| TEXAS INSTRUMENTS INCORPORATED
| Standard Linear and Logic Group
| IBIS Model of SN74AHC139
| DUAL 2-LINE TO 4-LINE DECODERS/DEMULTIPLEXERS
| This file contains package information for the following:
|  SOIC 16-pin (D) package as [Component] AHC139_D
|  SSOP 16-pin (DB) package as [Component] AHC139_DB
|  TVSOP 16-pin (DGV) package as [Component] AHC139_DGV
|  PDIP 16-pin (N) package as [Component] AHC139_N
|  SOP 16-pin (NS) package as [Component] AHC139_NS
|  TSSOP 16-pin (PW) package as [Component] AHC139_PW
|  QFN 16-pin (RGY) package as [Component] AHC139_RGY
| This device can be powered at the following Vccs:
|  5 volt Vcc
|  3.3 volt Vcc
| This file provides unique models under the [Model Selector] for each Vcc.
| For operation at a specific Vcc, select the appropriate model after each
| [Model Selector] keyword.
[IBIS Ver]   3.2
[Comment char]  |_char
[File Name]   sn74ahc139.ibs
[File Rev]   1.1 | X_die
[Date]   May 23, 2005
[Source]   Data created from TI-SPICE simulations at TI-SLL.
[Notes]   The following is an IBIS list for the AHC139.
   Please contact sllibis@ti.com with questions and
   comments concerning SLL IBIS models.
   This IBIS model is created from a BA (back annotated netlist)
   - FILE REV HISTORY
   - 1.1 Release IBIS file on 06/20/05
   - C_comp values are taken at a different test condition
   than the data sheet.
   - Power clamp data deleted as there is no power-clamp diode.
[Disclaimer] Property of Texas Instruments Incorporated.  Unauthorized
   reproduction and/or distribution is strictly prohibited.
   This product is protected under copyright law.
   Created  2005, (C) Copyright  2005, Texas Instruments
   Incorporated, All Rights Reserved
   UNLESS THERE IS A SIGNED, WRITTEN AGREEMENT TO THE
   CONTRARY, TEXAS INSTRUMENTS (TI) IS PROVIDING THE IBIS
   MODELS  AND WITHOUT ANY WARRANTY, EXPRESSED OR
   IMPLIED.  TI assumes no liability for:
   1) the accuracy of the IBIS models provided to your
   company;
   2) the proper functioning of these IBIS Models in your
   design or for any resulting applications; or
   3) infringement of patents, copyrights or intellectual
   property rights resulting from your use of these IBIS
   models.
   TI provides IBIS Models as a service to our customers.
   You and your company shall not distribute, sell or give
   these models to anyone else without prior written
   permission from TI.
   TI reserves the right to make changes to our products or
   to discontinue any semiconductor product or service
   without notice, and advises our customers to obtain the
   latest version of relevant information to verify, before
   placing orders, that the information being relied on is
   current.
   Please be aware that your receipt and use of the IBIS
   information provided shall serve as acceptance of these
   terms and conditions.  If you do not accept these terms,
   you should return or destroy the IBIS models and any
   other accompanying information immediately.
| Component ahc139_D 16-pin SOIC
[Component]   ahc139_D
[Manufacturer]   Texas Instruments, Inc.
[Package]
|   typ   min   max
R_pkg   3.900e-02   2.800e-02   4.900e-02
L_pkg   3.453e-09   2.350e-09   4.375e-09
C_pkg   5.210e-13   2.540e-13   7.080e-13
[Pin]   signal_name   model_name   R_pin   L_pin   C_pin
1   1NG   AHC139_ENABLE   4.200e-02   4.336e-09   7.030e-13
2   1A   AHC139_SELECT   4.900e-02   3.778e-09   6.340e-13
3   1B   AHC139_SELECT   2.800e-02   3.449e-09   5.180e-13
4   1Y0   AHC139_OUT   2.900e-02   2.393e-09   2.540e-13
5   1Y1   AHC139_OUT   2.800e-02   2.350e-09   2.640e-13
6   1Y2   AHC139_OUT   4.800e-02   3.312e-09   4.830e-13
7   1Y3   AHC139_OUT   4.300e-02   3.629e-09   6.040e-13
8   GND   GND   4.400e-02   4.375e-09   7.080e-13
9   2Y3   AHC139_OUT   4.200e-02   4.336e-09   7.030e-13
10   2Y2   AHC139_OUT   4.900e-02   3.778e-09   6.340e-13
11   2Y1   AHC139_OUT   2.800e-02   3.449e-09   5.180e-13
12   2Y0   AHC139_OUT   2.900e-02   2.393e-09   2.550e-13
13   2B   AHC139_SELECT   2.800e-02   2.350e-09   2.640e-13
14   2A   AHC139_SELECT   4.800e-02   3.312e-09   4.830e-13
15   2NG   AHC139_ENABLE   4.300e-02   3.629e-09   6.040e-13
16   VCC   POWER   4.400e-02   4.375e-09   7.080e-13
| Component ahc139_DB 16-pin SSOP
[Component]   ahc139_DB
[Manufacturer]   Texas Instruments, Inc.
[Package]
|   typ   min   max
R_pkg   4.800e-02   4.600e-02   5.000e-02
L_pkg   3.536e-09   3.213e-09   3.798e-09
C_pkg   3.760e-13   3.140e-13   4.400e-13
[Pin]   signal_name   model_name   R_pin   L_pin   C_pin
1   1NG   AHC139_ENABLE   4.800e-02   3.797e-09   3.770e-13
2   1A   AHC139_SELECT   4.600e-02   3.723e-09   4.400e-13
3   1B   AHC139_SELECT   4.800e-02   3.409e-09   3.720e-13
4   1Y0   AHC139_OUT   4.900e-02   3.213e-09   3.140e-13
5   1Y1   AHC139_OUT   4.900e-02   3.213e-09   3.140e-13
6   1Y2   AHC139_OUT   4.800e-02   3.409e-09   3.720e-13
7   1Y3   AHC139_OUT   4.600e-02   3.723e-09   4.400e-13
8   GND   GND   4.800e-02   3.798e-09   3.770e-13
9   2Y3   AHC139_OUT   4.800e-02   3.797e-09   3.770e-13
10   2Y2   AHC139_OUT   4.600e-02   3.725e-09   4.400e-13
11   2Y1   AHC139_OUT   4.800e-02   3.409e-09   3.720e-13
12   2Y0   AHC139_OUT   4.900e-02   3.214e-09   3.140e-13
13   2B   AHC139_SELECT   5.000e-02   3.216e-09   3.140e-13
14   2A   AHC139_SELECT   4.800e-02   3.409e-09   3.720e-13
15   2NG   AHC139_ENABLE   4.700e-02   3.729e-09   4.400e-13
16   VCC   POWER   4.800e-02   3.797e-09   3.770e-13
| Component ahc139_DGV 16-pin TVSOP
[Component]   ahc139_DGV
[Manufacturer]   Texas Instruments, Inc.
[Package]
|   typ   min   max
R_pkg   3.900e-02   3.300e-02   4.500e-02
L_pkg   2.543e-09   2.320e-09   2.938e-09
C_pkg   3.860e-13   3.340e-13   4.490e-13
[Pin]   signal_name   model_name   R_pin   L_pin   C_pin
1   1NG   AHC139_ENABLE   3.500e-02   2.907e-09   4.170e-13
2   1A   AHC139_SELECT   4.200e-02   2.558e-09   4.460e-13
3   1B   AHC139_SELECT   3.800e-02   2.341e-09   3.450e-13
4   1Y0   AHC139_OUT   3.800e-02   2.320e-09   3.340e-13
5   1Y1   AHC139_OUT   3.900e-02   2.322e-09   3.340e-13
6   1Y2   AHC139_OUT   3.800e-02   2.353e-09   3.420e-13
7   1Y3   AHC139_OUT   4.000e-02   2.536e-09   4.410e-13
8   GND   GND   3.300e-02   2.897e-09   4.180e-13
9   2Y3   AHC139_OUT   3.500e-02   2.927e-09   4.190e-13
10   2Y2   AHC139_OUT   4.500e-02   2.632e-09   4.490e-13
11   2Y1   AHC139_OUT   3.900e-02   2.368e-09   3.470e-13
12   2Y0   AHC139_OUT   3.900e-02   2.330e-09   3.350e-13
13   2B   AHC139_SELECT   3.900e-02   2.320e-09   3.350e-13
14   2A   AHC139_SELECT   3.900e-02   2.361e-09   3.450e-13
15   2NG   AHC139_ENABLE   4.100e-02   2.573e-09   4.460e-13
16   VCC   POWER   3.500e-02   2.938e-09   4.200e-13
| Component ahc139_N 16-pin PDIP
[Component]   ahc139_N
[Manufacturer]   Texas Instruments, Inc.
[Package]
|   typ   min   max
R_pkg   5.600e-02   5.200e-02   6.300e-02
L_pkg   7.637e-09   5.451e-09   1.053e-08
C_pkg   5.280e-13   3.350e-13   8.930e-13
[Pin]   signal_name   model_name   R_pin   L_pin   C_pin
1   1NG   AHC139_ENABLE   5.800e-02   1.053e-08   8.920e-13
2   1A   AHC139_SELECT   6.200e-02   8.759e-09   5.350e-13
3   1B   AHC139_SELECT   5.200e-02   7.146e-09   3.870e-13
4   1Y0   AHC139_OUT   5.300e-02   5.451e-09   4.080e-13
5   1Y1   AHC139_OUT   5.300e-02   5.513e-09   3.700e-13
6   1Y2   AHC139_OUT   5.300e-02   6.304e-09   3.360e-13
7   1Y3   AHC139_OUT   5.700e-02   7.830e-09   5.030e-13
8   GND   GND   5.600e-02   9.581e-09   8.050e-13
9   2Y3   AHC139_OUT   5.800e-02   9.603e-09   8.070e-13
10   2Y2   AHC139_OUT   6.200e-02   7.864e-09   5.030e-13
11   2Y1   AHC139_OUT   5.200e-02   6.295e-09   3.350e-13
12   2Y0   AHC139_OUT   5.300e-02   5.499e-09   3.560e-13
13   2B   AHC139_SELECT   5.300e-02   5.452e-09   4.040e-13
14   2A   AHC139_SELECT   5.300e-02   7.156e-09   3.870e-13
15   2NG   AHC139_ENABLE   6.300e-02   8.740e-09   5.340e-13
16   VCC   POWER   5.600e-02   1.048e-08   8.930e-13
| Component ahc139_NS 16-pin SOP
[Component]   ahc139_NS
[Manufacturer]   Texas Instruments, Inc.
[Package]
|   typ   min   max
R_pkg   4.200e-02   3.500e-02   4.900e-02
L_pkg   3.147e-09   2.164e-09   4.219e-09
C_pkg   4.040e-13   2.410e-13   5.620e-13
[Pin]   signal_name   model_name   R_pin   L_pin   C_pin
1   1NG   AHC139_ENABLE   4.900e-02   4.215e-09   5.620e-13
2   1A   AHC139_SELECT   4.600e-02   3.675e-09   4.800e-13
3   1B   AHC139_SELECT   3.700e-02   2.527e-09   3.320e-13
4   1Y0   AHC139_OUT   3.500e-02   2.164e-09   2.410e-13
5   1Y1   AHC139_OUT   3.500e-02   2.164e-09   2.410e-13
6   1Y2   AHC139_OUT   3.700e-02   2.527e-09   3.320e-13
7   1Y3   AHC139_OUT   4.600e-02   3.675e-09   4.800e-13
8   GND   GND   4.900e-02   4.215e-09   5.620e-13
9   2Y3   AHC139_OUT   4.900e-02   4.219e-09   5.620e-13
10   2Y2   AHC139_OUT   4.600e-02   3.679e-09   4.800e-13
11   2Y1   AHC139_OUT   3.700e-02   2.531e-09   3.330e-13
12   2Y0   AHC139_OUT   3.500e-02   2.168e-09   2.410e-13
13   2B   AHC139_SELECT   3.500e-02   2.168e-09   2.410e-13
14   2A   AHC139_SELECT   3.700e-02   2.531e-09   3.330e-13
15   2NG   AHC139_ENABLE   4.600e-02   3.679e-09   4.800e-13
16   VCC   POWER   4.900e-02   4.219e-09   5.620e-13
| Component AHC139_PW 16-pin TSSOP
[Component]   AHC139_PW
[Manufacturer]   Texas Instruments, Inc.
[Package]
|   typ   min   max
R_pkg   4.500e-02   3.800e-02   5.100e-02
L_pkg   2.593e-09   2.447e-09   3.080e-09
C_pkg   2.810e-13   2.430e-13   3.770e-13
[Pin]   signal_name   model_name   R_pin   L_pin   C_pin
1   1NG   AHC139_ENABLE   4.000e-02   3.080e-09   3.770e-13
2   1A   AHC139_SELECT   3.800e-02   2.458e-09   2.810e-13
3   1B   AHC139_SELECT   5.100e-02   2.512e-09   2.550e-13
4   1Y0   AHC139_OUT   5.100e-02   2.447e-09   2.430e-13
5   1Y1   AHC139_OUT   5.100e-02   2.447e-09   2.430e-13
6   1Y2   AHC139_OUT   5.100e-02   2.512e-09   2.550e-13
7   1Y3   AHC139_OUT   3.800e-02   2.458e-09   2.810e-13
8   GND   GND   4.000e-02   3.080e-09   3.770e-13
9   2Y3   AHC139_OUT   3.900e-02   2.832e-09   3.160e-13
10   2Y2   AHC139_OUT   3.800e-02   2.460e-09   2.790e-13
11   2Y1   AHC139_OUT   5.100e-02   2.512e-09   2.550e-13
12   2Y0   AHC139_OUT   5.100e-02   2.447e-09   2.430e-13
13   2B   AHC139_SELECT   5.100e-02   2.447e-09   2.430e-13
14   2A   AHC139_SELECT   5.100e-02   2.512e-09   2.550e-13
15   2NG   AHC139_ENABLE   3.800e-02   2.459e-09   2.790e-13
16   VCC   POWER   3.900e-02   2.832e-09   3.160e-13
| Component AHC139_RGY 16-pin QFN
[Component]   AHC139_RGY
[Manufacturer]   Texas Instruments, Inc.
[Package]
|   typ   min   max
R_pkg   3.900e-02   3.700e-02   4.200e-02
L_pkg   8.860e-10   8.430e-10   9.330e-10
C_pkg   3.270e-13   3.140e-13   3.360e-13
[Pin]   signal_name   model_name   R_pin   L_pin   C_pin
1   1NG   AHC139_ENABLE   4.100e-02   9.250e-10   3.140e-13
2   1A   AHC139_SELECT   4.000e-02   9.000e-10   3.260e-13
3   1B   AHC139_SELECT   3.900e-02   8.820e-10   3.330e-13
4   1Y0   AHC139_OUT   4.100e-02   9.150e-10   3.300e-13
5   1Y1   AHC139_OUT   4.000e-02   9.000e-10   3.300e-13
6   1Y2   AHC139_OUT   4.000e-02   8.910e-10   3.290e-13
7   1Y3   AHC139_OUT   4.100e-02   9.240e-10   3.300e-13
8   GND   GND   4.200e-02   9.330e-10   3.360e-13
9   2Y3   AHC139_OUT   3.900e-02   8.850e-10   3.250e-13
10   2Y2   AHC139_OUT   3.700e-02   8.430e-10   3.210e-13
11   2Y1   AHC139_OUT   3.900e-02   8.730e-10   3.310e-13
12   2Y0   AHC139_OUT   3.800e-02   8.550e-10   3.250e-13
13   2B   AHC139_SELECT   3.800e-02   8.530e-10   3.260e-13
14   2A   AHC139_SELECT   3.800e-02   8.570e-10   3.270e-13
15   2NG   AHC139_ENABLE   3.800e-02   8.540e-10   3.250e-13
16   VCC   POWER   3.900e-02   8.850e-10   3.190e-13
| Model AHC139_ENABLE
[Model Selector]   AHC139_ENABLE
AHC139_ENABLE_50   5 volt Vcc
AHC139_ENABLE_33   3.3 volt Vcc
| Model AHC139_SELECT
[Model Selector]   AHC139_SELECT
AHC139_SELECT_50   5 volt Vcc
AHC139_SELECT_33   3.3 volt Vcc
| Model AHC139_OUT
[Model Selector]   AHC139_OUT
AHC139_OUT_50   5 volt Vcc
AHC139_OUT_33   3.3 volt Vcc
| Models and submodels in the file (6): AHC139_ENABLE_50 (Input), AHC139_ENABLE_33 (Input), AHC139_SELECT_50 (Input), AHC139_SELECT_33 (Input), AHC139_OUT_50 (Output), AHC139_OUT_33 (Output)
